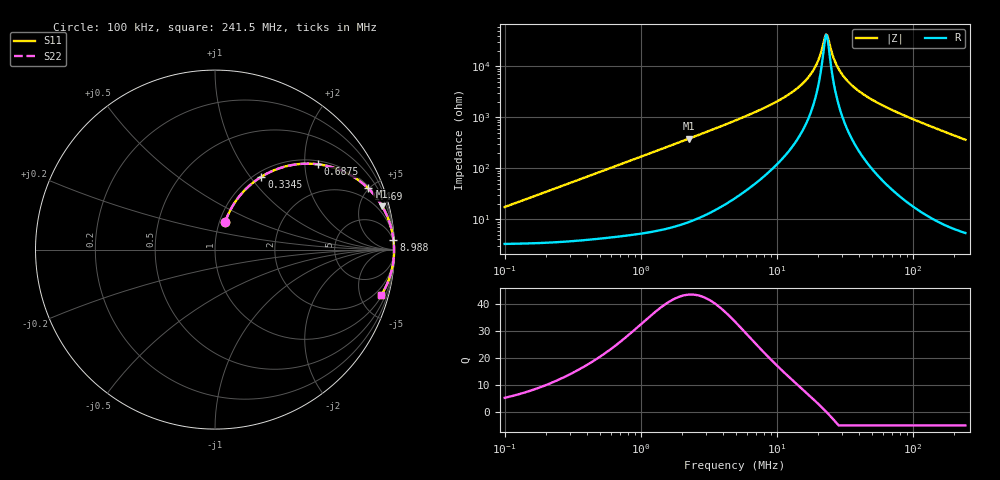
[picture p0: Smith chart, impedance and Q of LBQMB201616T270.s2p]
! LBQMB201616T270  S-PARAMETER MODEL  ( General Type )
! Model Generated by TAIYO YUDEN Corporation (http://www.ty-top.com)
! Version 1.0
! TAIYO YUDEN Control No. 191025NI43SB-FBB
! Copyright(c) 2019 TAIYO YUDEN CO.,LTD. All Rights Reserved.
! Product Description (link to TY-COMPAS)
! https://ds.yuden.co.jp/TYCOMPAS/or/detail?pn=LBQMB201616T270J&u=M
! Products Name : Inductors
! Characteristics :
!  Inductance : 27 uH , SRF(min) : 16 MHz , DC Resistance(max) : 4.16 Ohm , Rated Current : 130 mA
!  Case Size : 2.0 x 1.6 / 0.079 x 0.063 [mm/inch] , Thickness : 1.6 / 0.063 [mm/inch]
!  (Conditions: Temperature = 25 degC , DC Bias Current/Voltage = 0A / 0V)
! External Node Assignments :
!  1  o---GGG---o  2
! GND o---------o GND
! Frequency Range : 0.1MHz  -  241.513628MHz  [ 402 STEP ]
# MHz S RI R 50
! Freq[MHz].  S11 Real  S11 Imag  S21 Real  S21 Imag  S12 Real  S12 Imag  S22 Real  S22 Imag
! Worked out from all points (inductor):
!   401 points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, 100 kHz to 241.5 MHz, reference 50 ohm
!   read as one part in series: L = 27.2 uH near 104 kHz
!   highest Q = 43.4 at 2.255 MHz (marker M1), where L = 27 uH
!   self-resonance near 22.89 MHz
!   S11 on the Smith chart (normalised r, x): 100 kHz: 1.07, +0.34; 334.5 kHz: 1.08, +1.14; 687.5 kHz: 1.09, +2.32; 1.469 MHz: 1.13, +4.96; 8.988 MHz: 3, +35; 241.5 MHz: 1.11, -7.27
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0.1  0.0574 0.1558  0.9426 -0.1558  0.9426 -0.1558  0.0574 0.1558
0.193888  0.1227 0.2803  0.8773 -0.2803  0.8773 -0.2803  0.1227 0.2803
0.334469  0.2587 0.4061  0.7413 -0.4061  0.7413 -0.4061  0.2587 0.4061
0.368674  0.2937 0.4258  0.7063 -0.4258  0.7063 -0.4258  0.2937 0.4258
0.687508  0.5721 0.4755  0.4279 -0.4755  0.4279 -0.4755  0.5721 0.4755
1.359207  0.834 0.3592  0.166 -0.3592  0.166 -0.3592  0.834 0.3592
1.469315  0.8541 0.3406  0.1459 -0.3406  0.1459 -0.3406  0.8541 0.3406
2.255156  0.9312 0.2419  0.0688 -0.2419  0.0688 -0.2419  0.9312 0.2419
4.914404  0.9835 0.1134  0.0165 -0.1134  0.0165 -0.1134  0.9835 0.1134
8.987705  0.994 0.0558  0.00602 -0.0558  0.00602 -0.0558  0.994 0.0558
13.79465  0.9966 0.0277  0.0034 -0.0277  0.0034 -0.0277  0.9966 0.0277
16.12016  0.9971 0.0189  0.0029 -0.0189  0.0029 -0.0189  0.9971 0.0189
18.11814  0.9974 0.0126  0.00263 -0.0126  0.00263 -0.0126  0.9974 0.0126
19.97102  0.9975 0.00743  0.00246 -0.00743  0.00246 -0.00743  0.9975 0.00743
22.44628  0.9977 0.00133  0.00234 -0.00133  0.00234 -0.00133  0.9977 0.00133
23.33776  0.9977 -0.000691  0.00231 0.000691  0.00231 0.000691  0.9977 -0.000691
27.27206  0.9977 -0.00886  0.00229 0.00886  0.00229 0.00886  0.9977 -0.00886
29.48135  0.9977 -0.013  0.00234 0.013  0.00234 0.013  0.9977 -0.013
32.49632  0.9975 -0.0183  0.00245 0.0183  0.00245 0.0183  0.9975 -0.0183
43.52056  0.9967 -0.0356  0.00326 0.0356  0.00326 0.0356  0.9967 -0.0356
66.79689  0.9936 -0.0669  0.00643 0.0669  0.00643 0.0669  0.9936 -0.0669
241.5136  0.9264 -0.2538  0.0736 0.2538  0.0736 0.2538  0.9264 -0.2538
